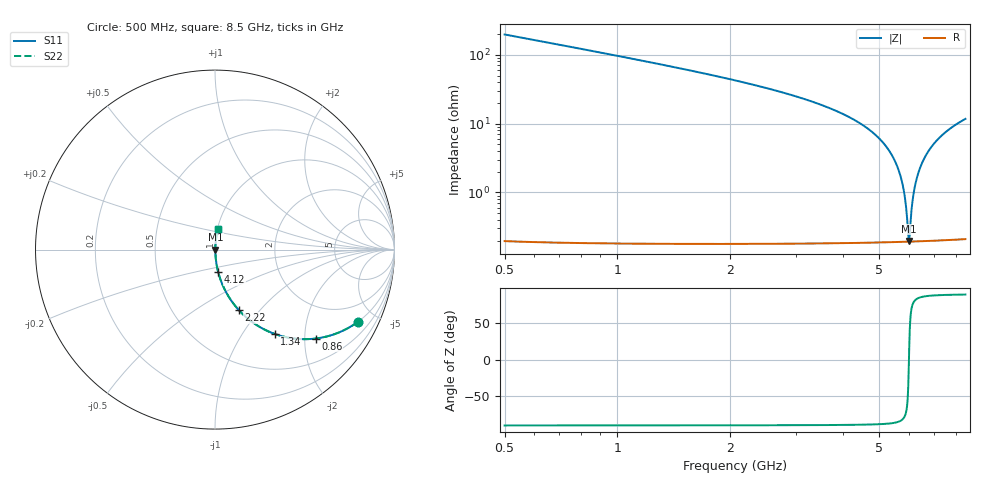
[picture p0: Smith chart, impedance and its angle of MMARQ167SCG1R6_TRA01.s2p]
! MMARQ167SCG1R6_TRA01  S-PARAMETER MODEL  ( General Type )
! Model Generated by TAIYO YUDEN Corporation (http://www.ty-top.com)
! Version 1.0
! TAIYO YUDEN Control No. 160201
! Copyright(c) 2016 TAIYO YUDEN CO.,LTD. All Rights Reserved.
! Product Description (link to TY-COMPAS)
! https://ds.yuden.co.jp/TYCOMPAS/or/detail?pn=MMARQ167SCG1R6BTRA01&u=M
! Products Name : Multilayer Ceramic Capacitors
! Characteristics :
!  Capacitance : 1.6 pF , Rated Voltage : 250V , TCC : CG / C0G
!  Case Size : 1.6 x 0.8 / 0.063 x 0.031 [mm/inch] , Thickness : 0.7 / 0.028 [mm/inch]
!  (Conditions: Temperature = 25 degC , DC Bias Current/Voltage = 0A / 0V)
! External Node Assignments :
!  1  o---| |---o  2
! GND o---------o GND
! Frequency Range : 500MHz  -  8500MHz  [ 401 STEP ]
# MHz S RI R 50
! Freq[MHz].  S11 Real  S11 Imag  S21 Real  S21 Imag  S12 Real  S12 Imag  S22 Real  S22 Imag
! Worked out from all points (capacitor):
!   401 points, 500 MHz to 8.5 GHz, reference 50 ohm
!   read as one part in series: C = 1.6 pF near 540 MHz
!   lowest |Z| = 197 mohm at 6 GHz (marker M1)
!   series resonance near 6.007 GHz, so ESL is about 440 pH
!   S11 on the Smith chart (normalised r, x): 500 MHz: 1.00, -3.95; 860 MHz: 1.00, -2.27; 1.34 GHz: 1.00, -1.41; 2.22 GHz: 1.00, -0.77; 4.12 GHz: 1.00, -0.26; 8.5 GHz: 1.00, +0.23
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500  0.7958 -0.4026  0.2042 0.4026  0.2042 0.4026  0.7958 -0.4026
860  0.562 -0.4953  0.438 0.4953  0.438 0.4953  0.562 -0.4953
1340  0.3326 -0.4699  0.6674 0.4699  0.6674 0.4699  0.3326 -0.4699
1840  0.1944 -0.3939  0.8056 0.3939  0.8056 0.3939  0.1944 -0.3939
2220  0.1313 -0.3355  0.8687 0.3355  0.8687 0.3355  0.1313 -0.3355
3180  0.0498 -0.2135  0.9502 0.2135  0.9502 0.2135  0.0498 -0.2135
4120  0.0178 -0.1254  0.9822 0.1254  0.9822 0.1254  0.0178 -0.1254
4500  0.0111 -0.0958  0.9889 0.0958  0.9889 0.0958  0.0111 -0.0958
5020  0.00541 -0.0593  0.9946 0.0593  0.9946 0.0593  0.00541 -0.0593
5400  0.00313 -0.0352  0.9969 0.0352  0.9969 0.0352  0.00313 -0.0352
5660  0.00229 -0.0197  0.9977 0.0197  0.9977 0.0197  0.00229 -0.0197
5840  0.002 -0.00932  0.998 0.00932  0.998 0.00932  0.002 -0.00932
5900  0.00195 -0.00595  0.998 0.00595  0.998 0.00595  0.00195 -0.00595
5980  0.00192 -0.00151  0.9981 0.00151  0.9981 0.00151  0.00192 -0.00151
6000  0.00192 -0.000408  0.9981 0.000408  0.9981 0.000408  0.00192 -0.000408
6040  0.00193 0.00178  0.9981 -0.00178  0.9981 -0.00178  0.00193 0.00178
6120  0.00197 0.00612  0.998 -0.00612  0.998 -0.00612  0.00197 0.00612
6180  0.00202 0.00934  0.998 -0.00934  0.998 -0.00934  0.00202 0.00934
6360  0.0023 0.0188  0.9977 -0.0188  0.9977 -0.0188  0.0023 0.0188
6680  0.00319 0.035  0.9968 -0.035  0.9968 -0.035  0.00319 0.035
7180  0.00549 0.0589  0.9945 -0.0589  0.9945 -0.0589  0.00549 0.0589
8500  0.0156 0.1152  0.9844 -0.1152  0.9844 -0.1152  0.0156 0.1152
